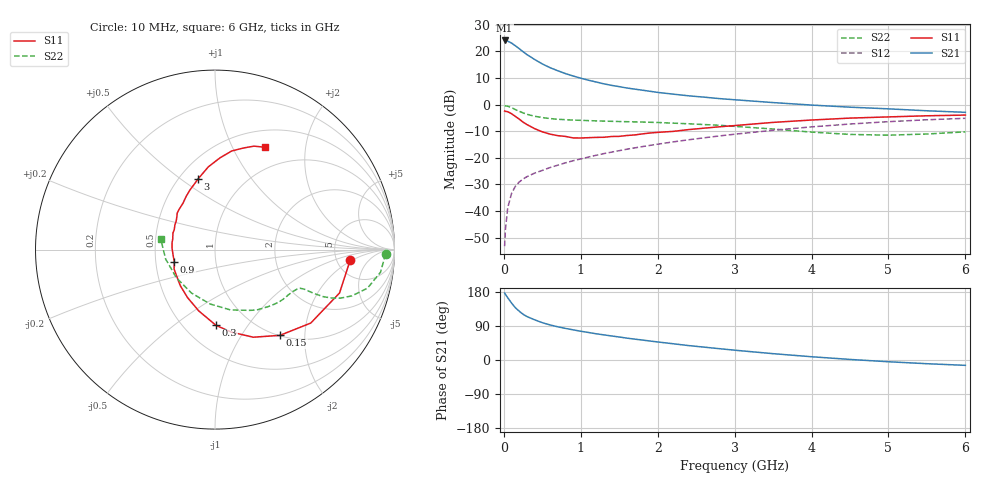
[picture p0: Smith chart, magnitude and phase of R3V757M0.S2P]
! SIEMENS Small Signal Semiconductors
! BFR181
! Si NPN RF Bipolar Junction Transistor in SOT23
! VCE = 0.75 V  IC = 7 mA
! Common Emitter S-Parameters:  May  1996
# GHz  S  MA  R  50
!  f  S11  S21  S12  S22
! GHz  MAG  ANG  MAG  ANG  MAG  ANG  MAG  ANG
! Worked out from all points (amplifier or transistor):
!   36 points, 10 MHz to 6 GHz, reference 50 ohm
!   highest |S21| = 24.1 dB at 10 MHz (marker M1)
!   |S21| within 3 dB of that: start of sweep to 196.6 MHz
!   unconditionally stable (mu >= 1): 520.5 MHz to 4.13 GHz; 5.901 GHz to end of sweep
!   at 250 MHz: K = 0.64, MSG = 23.9 dB, |S12| = -28.0 dB
!   at 1.4 GHz: K = 1.25, MAG = 9.5 dB, |S12| = -17.9 dB
!   at 6 GHz: K = 1.00, MAG = 0.8 dB, |S12| = -5.2 dB
!   S11 on the Smith chart (normalised r, x): 10 MHz: 6.72, -1.78; 150 MHz: 1.01, -1.50; 300 MHz: 0.70, -0.72; 900 MHz: 0.63, -0.09; 3 GHz: 0.62, +0.58; 6 GHz: 0.71, +1.35
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0.01  0.7562 -4.3  15.96 176.8  0.0022 85.9  0.9525 -1.5
0.02  0.7461 -7.9  15.82 173.4  0.0044 84.7  0.9441 -3.2
0.05  0.7347 -19.2  15.49 164.4  0.0115 78.6  0.9307 -7.8
0.1  0.6724 -37.5  14.26 150.4  0.0214 73.1  0.8764 -14.2
0.15  0.5991 -52.9  12.67 137.9  0.0293 66.2  0.8046 -18.7
0.2  0.5327 -66.4  11.2 128.8  0.0352 63.0  0.7486 -21.2
0.25  0.4678 -79.0  9.806 120.7  0.04 60.3  0.6976 -22.7
0.3  0.4216 -89.3  8.669 114.7  0.0443 59.2  0.6565 -23.5
0.4  0.3532 -104.9  7.025 106.1  0.0517 59.1  0.6033 -23.9
0.5  0.3078 -119.9  5.782 98.5  0.0581 59.7  0.57 -23.9
0.6  0.2787 -134.0  4.932 92.6  0.0657 60.7  0.5462 -23.9
0.7  0.2608 -144.5  4.314 87.6  0.0728 61.5  0.5295 -24.2
0.9  0.2369 -163.4  3.438 79.6  0.0882 62.8  0.5118 -25.2
1.1  0.239 178.7  2.866 72.6  0.1035 63.9  0.4998 -27.0
1.3  0.243 165.3  2.448 66.3  0.1201 63.8  0.4892 -29.1
1.6  0.2627 148.2  2.043 57.7  0.1453 63.7  0.4769 -33.0
2.2  0.3136 124.8  1.569 42.9  0.1992 60.9  0.4479 -43.0
3  0.4031 103.8  1.231 25.9  0.2775 54.5  0.3901 -60.2
3.5  0.4626 94.6  1.089 16.7  0.329 49.3  0.3471 -75.6
4.5  0.5572 80.4  0.893 1.5  0.4311 36.8  0.2751 -118.6
5.5  0.6157 69.4  0.764 -9.8  0.5181 22.7  0.2801 -169.2
6  0.6347 64.0  0.715 -14.1  0.5521 15.4  0.3074 169.2
